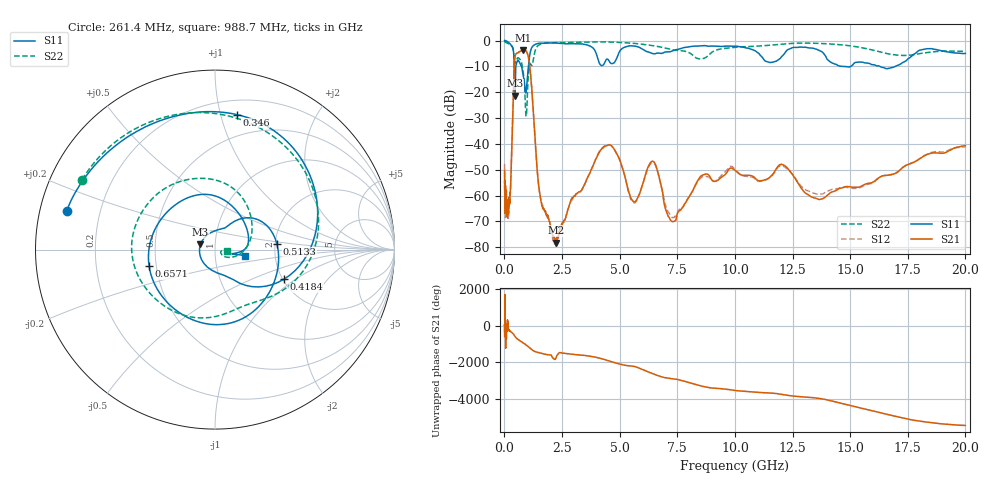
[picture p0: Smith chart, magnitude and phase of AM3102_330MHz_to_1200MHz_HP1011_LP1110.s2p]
! Date/Time: Tue, Sep 11, 2018 5:20 PM
! Network Analyzer: Agilent Technologies E8362B Rev: A.07.50.63
! Sweep from 0.010 to 20.000 GHz, 1601 Points, Sweep Type: LOG
! Power Supply: 4.949 V, 0.001 A
# Hz S DB R 50
!freq MagS11 AngS11 MagS21 AngS21 MagS12 AngS12 MagS22 AngS22
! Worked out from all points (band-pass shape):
!   1601 points, 10 MHz to 20 GHz, reference 50 ohm
!   highest |S21| = -3.67 dB at 821.5 MHz (marker M1); lowest = -78.2 dB at 2.228 GHz (marker M2)
!   |S21| within 3 dB of the highest: 453 MHz to 1.047 GHz (594.1 MHz wide, 79.2 % of centre)
!   lowest |S11| = -21.3 dB at 455.8 MHz (marker M3), VSWR 1.19, Z = 42.4 + j2.44 ohm
!   |S11| at or under -10 dB: 741.1 MHz to 1.043 GHz (301.9 MHz wide, 33.8 % of centre); 14.66 GHz to 15.02 GHz (361.2 MHz wide, 2.43 % of centre); 16.29 GHz to 16.96 GHz (672.9 MHz wide, 4.05 % of centre)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
!   |S22| runs from -29.3 to -0.2 dB; largest |S21 - S12| = 0.009
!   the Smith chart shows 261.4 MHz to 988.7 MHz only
!   S11 on the Smith chart (normalised r, x): 261.4 MHz: 0.08, +0.13; 346 MHz: 0.31, +1.12; 418.4 MHz: 2.03, -0.81; 513.3 MHz: 2.04, +0.16; 657.1 MHz: 0.46, -0.10; 988.7 MHz: 1.40, -0.10
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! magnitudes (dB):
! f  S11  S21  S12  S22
! 10 MHz  0.0  -50.2  -48.1  -0.2
! 35.55 MHz  0.0  -64.6  -64.2  -0.5
! 126.4 MHz  -0.4  -66.2  -66.2  -1.0
! 261.4 MHz  -1.4  -58.5  -58.3  -1.5
! 346 MHz  -2.4  -33.3  -33.4  -2.5
! 418.4 MHz  -7.6  -11.7  -11.7  -5.9
! 447.2 MHz  -20.6  -7.2  -7.2  -8.6
! 455.8 MHz  -21.3  -6.5  -6.5  -9.0
! 513.3 MHz  -9.2  -5.0  -5.1  -7.7
! 657.1 MHz  -8.4  -4.3  -4.4  -7.1
! 821.5 MHz  -13.8  -3.7  -3.7  -12.4
! 988.7 MHz  -15.3  -4.8  -4.8  -23.2
! 1.151 GHz  -3.6  -14.4  -14.5  -9.2
! 1.59 GHz  -1.0  -62.3  -61.9  -1.3
! 2.228 GHz  -0.9  -78.2  -79.2  -0.8
! 4.394 GHz  -7.7  -40.8  -40.7  -0.5
! 5.652 GHz  -2.1  -62.4  -62.9  -1.1
! 6.396 GHz  -4.9  -46.8  -47.3  -1.9
! 7.271 GHz  -4.1  -70.0  -68.4  -3.5
! 9.808 GHz  -2.2  -49.4  -48.7  -2.8
! 13.74 GHz  -4.2  -61.4  -59.4  -1.1
! 20 GHz  -5.0  -40.6  -41.2  -4.2
